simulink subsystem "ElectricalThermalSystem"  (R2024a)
settings: Solver=VariableStepAuto  StartTime=0.0  StopTime=10.0  RelTol=1e-3
undefined symbols (not defined in the file): EnvAirTemp, PlantThrEstCmpPwr, PlntThrAirBpt, PlntThrAirCond, PlntThrAirCp, PlntThrAirCpBpt, PlntThrAirPrand, PlntThrAirRho, PlntThrAirVisc, PlntThrBattDCFlwRatio, PlntThrBattJacLen, PlntThrChArea, PlntThrChDia, PlntThrCoolCond, PlntThrCoolCp, PlntThrCoolCpBpt, PlntThrCoolPrand, PlntThrCoolRho, PlntThrCoolVisc, PlntThrDCJacLen, PlntThrEMJacLen, PlntThrEstCOPLut, PlntThrEstDTLut, PlntThrHeaterMaxPwr, PlntThrPmpDisp, PlntThrPmpHeadP, PlntThrPmpMaxSpd, PlntThrPmpMechEff, PlntThrPmpVolEff, PlntThrRadAirArea, PlntThrRadAirDh, PlntThrRadFanAreaFlw, PlntThrRadFlwCoef, PlntThrRadGapHeight, PlntThrRadLength, PlntThrRadNTubes, PlntThrRadTubeDh, PlntThrRadTubeHeight, PlntThrRadWidth
libraries: autolibutils x45
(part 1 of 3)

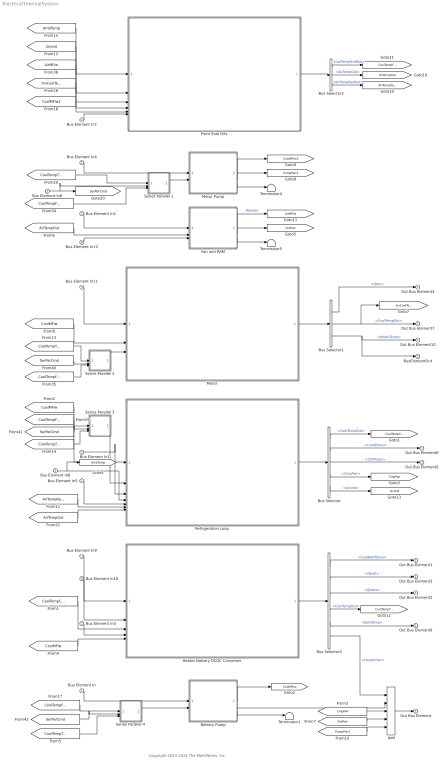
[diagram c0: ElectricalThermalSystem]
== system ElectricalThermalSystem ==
  note: Copyright 2023-2024 The MathWorks, Inc.
  Bus Element In{,1..7} (8 alike) : Inport
  Bus Element In8 : Inport  Port=2
  Bus Element In9 : Inport  Port=3
  Bus Element In10 : Inport  Port=4
  Bus Element In11 : Inport  Port=5
  Bus Element In12 : Inport  Port=6
  Add : Sum  Inputs=+++++
  Battery Pump : Subsystem  mask{DispAng=PlntThrPmpDisp, MaxSpd=PlntThrPmpMaxSpd, VolEff=PlntThrPmpVolEff, MechEff=PlntThrPmpMechEff, HeadP=PlntThrPmpHeadP}
      mask prompts: DispAng "Displacement per revolution, DispAng [L/rev]"; MaxSpd "Max angular speed, MaxSpd [rpm]"; VolEff "Volumetric efficiency, VolEff [-]"; MechEff "Mechanical efficiency, MechEff [-]"; HeadP "Pressure gain, HeadP [Pa]"
  Bus Selector : BusSelector  OutputSignals=CoolTempOut,CondPress,ChlrPress,CmpPwr,Qcond
  Bus Selector1 : BusSelector  OutputSignals=Qem,CoolTempOut,MotorTemp
  Bus Selector2 : BusSelector  OutputSignals=CoolTempFrmRad,AirTempOut,AirTempRadOut
  Bus Selector3 : BusSelector  OutputSignals=CoolBattTemp,Qbatt,Qpwre,CoolTempOut,BattTemp,HeaterPwr
  Fan and RAM : Subsystem  mask{DispAng=PlntThrPmpDisp, MaxSpd=PlntThrPmpMaxSpd, VolEff=PlntThrPmpVolEff, MechEff=PlntThrPmpMechEff, HeadP=PlntThrPmpHeadP}
      mask prompts: DispAng "Displacement per revolution, DispAng [L/rev]"; MaxSpd "Max angular speed, MaxSpd [rpm]"; VolEff "Volumetric efficiency, VolEff [-]"; MechEff "Mechanical efficiency, MechEff [-]"; HeadP "Pressure gain, HeadP [Pa]"
  Front Side HXs : Subsystem
  Heater Battery DCDC Converter : Subsystem
  Motor : Subsystem  Variant=on
  Motor Pump : Subsystem  mask{DispAng=PlntThrPmpDisp, MaxSpd=PlntThrPmpMaxSpd, VolEff=PlntThrPmpVolEff, MechEff=PlntThrPmpMechEff, HeadP=PlntThrPmpHeadP}
      mask prompts: DispAng "Displacement per revolution, DispAng [L/rev]"; MaxSpd "Max angular speed, MaxSpd [rpm]"; VolEff "Volumetric efficiency, VolEff [-]"; MechEff "Mechanical efficiency, MechEff [-]"; HeadP "Pressure gain, HeadP [Pa]"
  Refrigeration Loop : Subsystem
  Series Parallel 1 : Subsystem
  Series Parallel 2 : Subsystem
  Series Parallel 3 : Subsystem
  Series Parallel 4 : Subsystem
  Terminator1 : Terminator
  Terminator4 : Terminator
  Terminator5 : Terminator
  Out Bus Element{,1..7,9..10} (10 alike) : Outport
  BusElementOut : Outport
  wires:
  Bus Element In9/1 -> Heater Battery DCDC Converter/1(BattTemp)
  Bus Element In10/1 -> Heater Battery DCDC Converter/2(PwrETemp)
  Series Parallel 4/1(Out1) -> Battery Pump/2(FluidTemp)
  Series Parallel 3/1(Out1) -> Refrigeration Loop/2(CoolTempIn)
  Series Parallel 1/1(Out1) -> Motor Pump/2(FluidTemp)
  Motor/1(Info) -> Bus Selector1/1
  Series Parallel 2/1(Out1) -> Motor/3(CoolTempIn)
  [CoolMFlw] -> Motor/2(CoolMFlow)
  Bus Element In11/1 -> Motor/1(EMTemp)
  Bus Element In12/1 -> Fan and RAM/3(xdot)
  Bus Element In8/1 -> Refrigeration Loop/4(AmbTemp), [AmbTemp]
  [AirTempOut] -> Refrigeration Loop/7(AirTempCondOut)
  [AirTempRadOut] -> Refrigeration Loop/6(AirTempCondIn)
  Bus Selector2/3 -> [AirTempRadOut]  "<AirTempRadOut>"
  Bus Element In5/1 -> Refrigeration Loop/5(ByPCmd)
  Bus Element In7/1 -> Front Side HXs/6(ByPCmd)
  Bus Element In/1 -> Battery Pump/1(Cmd)
  Battery Pump/1(Mdot) -> [CoolMFlw]
  Battery Pump/3(Trq) -> Terminator1/1
  Bus Element In3/1 -> Heater Battery DCDC Converter/4(HeaterCmd)
  Heater Battery DCDC Converter/1(Bus Element Out) -> Bus Selector3/1
  Bus Selector3/1 -> Out Bus Element1/1  "<CoolBattTemp>"
  Bus Selector3/2 -> Out Bus Element3/1  "<Qbatt>"
  Bus Selector3/3 -> Out Bus Element2/1  "<Qpwre>"
  Bus Selector3/4 -> [CoolTempToRorC]  "<CoolTempOut>"
  [CoolMFlw] -> Refrigeration Loop/1(CoolMFlow)
  Bus Element In1/1 -> Refrigeration Loop/3(CmpCmd)
  [CoolTempChlrOut] -> Heater Battery DCDC Converter/3(CoolTempIn)
  Bus Selector/4 -> [CmpPwr]  "<CmpPwr>"
  Bus Selector/2 -> Out Bus Element6/1  "<CondPress>"
  Bus Selector/3 -> Out Bus Element5/1  "<ChlrPress>"
  Add/1 -> Out Bus Element/1
  [CoolMFlw] -> Heater Battery DCDC Converter/5(CoolMFlw)
  [AirTempOut] -> Fan and RAM/2(AirTemp)
  Bus Element In2/1 -> Fan and RAM/1(Cmd)
  Fan and RAM/1(Mdot) -> [AirMFlw]  "MdotAir"
  Fan and RAM/2(Pwr) -> [FanPwr]
  Fan and RAM/3(Trq) -> Terminator5/1
  Bus Selector1/1 -> Out Bus Element4/1  "<Qem>"
  Bus Selector1/2 -> Out Bus Element7/1, [InvCoolTempOut]  "<CoolTempOut>"
  Bus Element In4/1 -> Motor Pump/1(Cmd)
  Motor Pump/3(Trq) -> Terminator4/1
  Motor Pump/2(Pwr) -> [PumpPwr2]
  Motor Pump/1(Mdot) -> [CoolMFlw2]
  Bus Selector/5 -> [Qcond]  "<Qcond>"
  Refrigeration Loop/1(Out Bus Element) -> Bus Selector/1
  [AmbTemp] -> Front Side HXs/1(AmbTemp)
  [Qcond] -> Front Side HXs/2(Qcond)
  [AirMFlw] -> Front Side HXs/3(AirMFlw)
  [InvCoolTempOut] -> Front Side HXs/4(CoolTempToRad)
  Front Side HXs/1(Out Bus Element) -> Bus Selector2/1
  Bus Selector2/2 -> [AirTempOut]  "<AirTempOut>"
  [SerParCmd] -> Series Parallel 2/2(In2)
  [SerParCmd] -> Series Parallel 4/2(In2)
  [SerParCmd] -> Series Parallel 3/2(In2)
  Bus Element In6/1 -> [SerParCmd], Series Parallel 1/2(In2)
  [CoolMFlw2] -> Front Side HXs/5(CoolMFlw2)
  Bus Selector2/1 -> [CoolTempFrmRad]  "<CoolTempFrmRad>"
  Bus Selector/1 -> [CoolTempChlrOut]  "<CoolTempOut>"
  Bus Selector1/3 -> Out Bus Element10/1, BusElementOut/1  "<MotorTemp>"
  Bus Selector3/5 -> Out Bus Element9/1  "<BattTemp>"
  [PumpPwr2] -> Add/5
  [FanPwr] -> Add/4
  [CmpPwr] -> Add/3
  Battery Pump/2(Pwr) -> Add/2
  Bus Selector3/6 -> Add/1  "<HeaterPwr>"
  [CoolTempFrmRad] -> Series Parallel 3/1(In1)
  [CoolTempToRorC] -> Series Parallel 3/3(In3)
  [CoolTempToRorC] -> Series Parallel 2/1(In1)
  [CoolTempFrmRad] -> Series Parallel 2/3(In3)
  [CoolTempFrmRad] -> Series Parallel 4/1(In1)
  [CoolTempToRorC] -> Series Parallel 4/3(In3)
  [CoolTempToRorC] -> Series Parallel 1/1(In1)
  [CoolTempFrmRad] -> Series Parallel 1/3(In3)

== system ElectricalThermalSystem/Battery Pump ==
  Cmd : Inport
  FluidTemp : Inport  Port=2
  Density : Lookup_n-D  NumberOfTableDimensions=1  BreakpointsForDimension1=PlntThrCoolCpBpt  Table=PlntThrCoolRho  ExtrapMethod=Clip  UseLastTableValue=on  InternalRulePriority=Speed  RndMeth=Simplest
  Displ_LperRev : Constant  Value=DispAng  SampleTime=-1
  Gain : Gain  Gain=2*pi/60
  Gain1 : Gain  Gain=1/(1000*2*pi)
  LPF with IC1 : Subsystem  mask{wc=100, InitCond=0, dataType=off}
      mask prompts: wc "Cutoff frequency, wc [rad/s]"; InitCond "Initial condition, InitCond [same as u]"; dataType "Enforce same input data type"
  MaxSpd_rpm : Constant  Value=MaxSpd  SampleTime=-1
  MechanicalEfficiency : Constant  Value=MechEff  SampleTime=-1
  PressGain_Pa : Constant  Value=HeadP  SampleTime=-1
  Product : Product  Inputs=4
  Product1 : Product  Inputs=3
  Product2 : Product
  Product7 : Product
  Saturation : Saturate  UpperLimit=inf  LowerLimit=0
  VolumetricEfficiency : Constant  Value=VolEff  SampleTime=-1
  Mdot : Outport
  Pwr : Outport  Port=2
  Trq : Outport  Port=3
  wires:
  Saturation/1 -> Mdot/1
  LPF with IC1/1(y) -> Product7/2
  FluidTemp/1 -> Density/1
  VolumetricEfficiency/1 -> [VolEff]
  Density/1 -> Product/1
  MaxSpd_rpm/1 -> Gain/1
  Gain/1 -> Product7/1
  Displ_LperRev/1 -> Gain1/1
  Product7/1 -> [Spd]
  [Spd] -> Product/3
  [VolEff] -> Product/4
  MechanicalEfficiency/1 -> Product1/2
  [Spd] -> Product2/1
  PressGain_Pa/1 -> Product1/3
  Product1/1 -> Trq/1, Product2/2
  Gain1/1 -> Product1/1, Product/2
  Product/1 -> Saturation/1
  Cmd/1 -> LPF with IC1/1(u)
  Product2/1 -> Pwr/1

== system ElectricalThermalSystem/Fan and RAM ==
  Cmd : Inport
  AirTemp : Inport  Port=2
  xdot : Inport  Port=3
  Add : Sum
  Density : Lookup_n-D  NumberOfTableDimensions=1  BreakpointsForDimension1=PlntThrAirBpt  Table=PlntThrAirRho  ExtrapMethod=Clip  UseLastTableValue=on  InternalRulePriority=Speed  RndMeth=Simplest
  Displ_LperRev : Constant  Value=DispAng  SampleTime=-1
  Gain : Gain  Gain=PlntThrRadFanAreaFlw*PlntThrRadFlwCoef
  Gain1 : Gain  Gain=2*pi/60
  Gain2 : Gain  Gain=1/(1000*2*pi)
  LPF with IC1 : Subsystem  mask{wc=100, InitCond=0, dataType=off}
      mask prompts: wc "Cutoff frequency, wc [rad/s]"; InitCond "Initial condition, InitCond [same as u]"; dataType "Enforce same input data type"
  MaxSpd_rpm : Constant  Value=MaxSpd  SampleTime=-1
  MechanicalEfficiency : Constant  Value=MechEff  SampleTime=-1
  PressGain_Pa : Constant  Value=HeadP  SampleTime=-1
  Product : Product  Inputs=3
  Product1 : Product  Inputs=3
  Product2 : Product
  Product4 : Product
  Product7 : Product
  Saturation : Saturate  UpperLimit=inf  LowerLimit=0
  VolumetricEfficiency : Constant  Value=VolEff  SampleTime=-1
  Mdot : Outport
  Pwr : Outport  Port=2
  Trq : Outport  Port=3
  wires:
  Product4/1 -> Saturation/1
  Saturation/1 -> Mdot/1
  LPF with IC1/1(y) -> Product7/2
  AirTemp/1 -> Density/1
  Product/1 -> Add/2  "FanAir"
  xdot/1 -> Gain/1
  VolumetricEfficiency/1 -> [VolEff]
  Density/1 -> Product4/1
  MaxSpd_rpm/1 -> Gain1/1
  Gain1/1 -> Product7/1
  Displ_LperRev/1 -> Gain2/1
  Product7/1 -> [Spd]
  MechanicalEfficiency/1 -> Product1/2
  [Spd] -> Product2/1
  PressGain_Pa/1 -> Product1/3
  Product1/1 -> Trq/1, Product2/2
  Gain2/1 -> Product1/1, Product/1
  Cmd/1 -> LPF with IC1/1(u)
  Product2/1 -> Pwr/1
  [VolEff] -> Product/3
  [Spd] -> Product/2
  Add/1 -> Product4/2
  Gain/1 -> Add/1

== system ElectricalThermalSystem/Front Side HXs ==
  AmbTemp : Inport
  Qcond : Inport  Port=2
  AirMFlw : Inport  Port=3
  CoolTempToRad : Inport  Port=4
  CoolMFlw2 : Inport  Port=5
  ByPCmd : Inport  Port=6
  Condenser : Subsystem
  Radiator : Subsystem
  Out Bus Element{,1..3} (4 alike) : Outport
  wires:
  [AirMassFlw] -> Condenser/2(AirMassFlow)
  Radiator/2(Qrad) -> Out Bus Element2/1
  Radiator/1(CoolTempFrmRad) -> Out Bus Element/1
  ByPCmd/1 -> Radiator/5(ByPCmd)
  CoolMFlw2/1 -> Radiator/3(CoolMFlw)
  AmbTemp/1 -> Radiator/2(AmbTemp)
  CoolTempToRad/1 -> Radiator/1(CoolTempToRad)
  Radiator/3(AirTempOut) -> Out Bus Element3/1, Condenser/3(AirTempRadOut)
  Condenser/1(AirTempOut) -> Out Bus Element1/1
  Qcond/1 -> Condenser/1(Qcond)
  AirMFlw/1 -> [AirMassFlw], Radiator/4(MassFlow2)  "AirMassFlow"

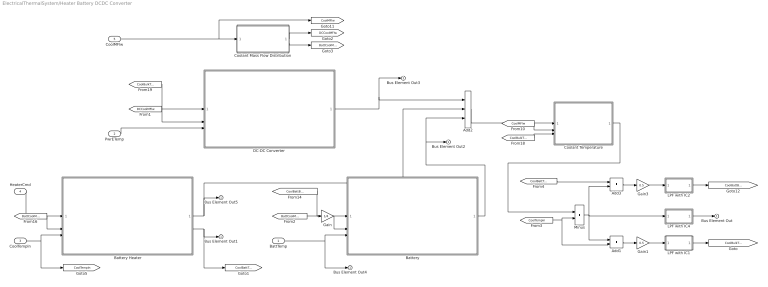
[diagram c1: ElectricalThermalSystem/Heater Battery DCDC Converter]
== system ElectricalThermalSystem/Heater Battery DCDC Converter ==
  BattTemp : Inport
  PwrETemp : Inport  Port=2
  CoolTempIn : Inport  Port=3
  HeaterCmd : Inport  Port=4
  CoolMFlw : Inport  Port=5
  Add1 : Sum
  Add2 : Sum  Inputs=+++
  Add3 : Sum
  Battery : Subsystem  mask{JacArea=PlntThrChArea, JacDia=PlntThrChDia, JacLen=PlntThrBattJacLen, JacHtArea=PlntThrBattJacLen*pi*PlntThrChDia}
      mask prompts: JacArea "Jacket cross section area, JacArea [m^2]"; JacDia "Jacket hydraulic diameter, JacDia [m]"; JacLen "Jacket length, JacLen [m]"; JacHtArea "Jacket heat transfer area, JacHtArea [m^2]"
  Battery Heater : Subsystem  mask{HtPwr=PlntThrHeaterMaxPwr}
      mask prompts: HtPwr "Maximum battery heater power, Gain [W]"
  Coolant Mass Flow Distribution : Subsystem  mask{MFlwRt=PlntThrBattDCFlwRatio}
      mask prompts: MFlwRt "Battery / DC-DC converter flow ratio, MFlwRt [-]"
  Coolant Temperature : Subsystem
  DC-DC Converter : Subsystem  mask{JacArea=PlntThrChArea, JacDia=PlntThrChDia, JacLen=PlntThrDCJacLen, JacHtArea=PlntThrDCJacLen*pi*PlntThrChDia}
      mask prompts: JacArea "Jacket cross section area, JacArea [m^2]"; JacDia "Jacket hydraulic diameter, JacDia [m]"; JacLen "Jacket length, JacLen [m]"; JacHtArea "Jacket heat transfer area, JacHtArea [m^2]"
  Gain : Gain  Gain=1/4
  Gain1 : Gain  Gain=0.5
  Gain3 : Gain  Gain=0.5
  LPF with IC1 : Subsystem  mask{wc=10, InitCond=EnvAirTemp, dataType=off}
      mask prompts: wc "Cutoff frequency, wc [rad/s]"; InitCond "Initial condition, InitCond [same as u]"; dataType "Enforce same input data type"
  LPF with IC2 : Subsystem  mask{wc=10, InitCond=EnvAirTemp, dataType=off}
      mask prompts: wc "Cutoff frequency, wc [rad/s]"; InitCond "Initial condition, InitCond [same as u]"; dataType "Enforce same input data type"
  LPF with IC4 : Subsystem  mask{wc=10, InitCond=EnvAirTemp, dataType=off}
      mask prompts: wc "Cutoff frequency, wc [rad/s]"; InitCond "Initial condition, InitCond [same as u]"; dataType "Enforce same input data type"
  Minus : Sum
  Bus Element Out{,1..5} (6 alike) : Outport
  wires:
  Battery Heater/1(Qheater) -> Add2/2, Bus Element Out5/1
  [CoolBattTempIn] -> Add3/1
  Battery Heater/2(CoolBattTemp) -> Bus Element Out1/1, [CoolBattTempIn]
  Coolant Temperature/1(DeltaTemp) -> Minus/1
  [CoolBulkTemp] -> Coolant Temperature/3(CoolBlkTemp)
  [CoolMFlw] -> Coolant Temperature/2(CoolMFlw)
  Add2/1 -> Coolant Temperature/1(Qsum)
  [BattCoolMFlw] -> Battery Heater/2(BattCoolMFlw)
  HeaterCmd/1 -> Battery Heater/1(HeaterCmd)
  PwrETemp/1 -> DC-DC Converter/3(PwrETemp)
  [DCCoolMFlw] -> DC-DC Converter/2(MassFlow)
  [CoolBulkTemp] -> DC-DC Converter/1(FluidTemp)
  DC-DC Converter/1(Qpwre) -> Add2/1, Bus Element Out3/1
  Gain/1 -> Battery/2(MassFlow)
  [CoolBattBulkTemp] -> Battery/1(FluidTemp)
  Battery/1(Qbatt) -> Bus Element Out2/1, Add2/3
  BattTemp/1 -> Bus Element Out4/1, Battery/3(BattTemp)
  Coolant Mass Flow Distribution/2(BattCoolMFlw) -> [BattCoolMFlw]
  Coolant Mass Flow Distribution/1(DCCoolMFlw) -> [DCCoolMFlw]
  [BattCoolMFlw] -> Gain/1
  LPF with IC4/1(y) -> Bus Element Out/1
  LPF with IC1/1(y) -> [CoolBulkTemp]
  Gain1/1 -> LPF with IC1/1(u)
  LPF with IC2/1(y) -> [CoolBattBulkTemp]
  Gain3/1 -> LPF with IC2/1(u)
  Add1/1 -> Gain1/1
  CoolTempIn/1 -> Battery Heater/3(CoolTempIn), [CoolTempIn]
  CoolMFlw/1 -> Coolant Mass Flow Distribution/1(CoolMFlw), [CoolMFlw]
  Add3/1 -> Gain3/1
  Minus/1 -> Add3/2, Add1/1, LPF with IC4/1(u)
  [CoolTempIn] -> Minus/2, Add1/2

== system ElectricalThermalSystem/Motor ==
  EMTemp : Inport
  CoolMFlow : Inport  Port=2
  CoolTempIn : Inport  Port=3
  FourEMs : Subsystem  VariantControl=PlntEMNum == 4
  OneEM : Subsystem  VariantControl=PlntEMNum == 1
  ThreeEMs : Subsystem  VariantControl=PlntEMNum == 3
  TwoEMs : Subsystem  VariantControl=PlntEMNum == 2
  Info : Outport

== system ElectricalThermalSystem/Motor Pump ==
  Cmd : Inport
  FluidTemp : Inport  Port=2
  Density : Lookup_n-D  NumberOfTableDimensions=1  BreakpointsForDimension1=PlntThrCoolCpBpt  Table=PlntThrCoolRho  ExtrapMethod=Clip  UseLastTableValue=on  InternalRulePriority=Speed  RndMeth=Simplest
  Displ_LperRev : Constant  Value=DispAng  SampleTime=-1
  Gain : Gain  Gain=2*pi/60
  Gain1 : Gain  Gain=1/(1000*2*pi)
  LPF with IC1 : Subsystem  mask{wc=100, InitCond=0, dataType=off}
      mask prompts: wc "Cutoff frequency, wc [rad/s]"; InitCond "Initial condition, InitCond [same as u]"; dataType "Enforce same input data type"
  MaxSpd_rpm : Constant  Value=MaxSpd  SampleTime=-1
  MechanicalEfficiency : Constant  Value=MechEff  SampleTime=-1
  PressGain_Pa : Constant  Value=HeadP  SampleTime=-1
  Product : Product  Inputs=4
  Product1 : Product  Inputs=3
  Product2 : Product
  Product7 : Product
  Saturation : Saturate  UpperLimit=inf  LowerLimit=0
  VolumetricEfficiency : Constant  Value=VolEff  SampleTime=-1
  Mdot : Outport
  Pwr : Outport  Port=2
  Trq : Outport  Port=3
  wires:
  Saturation/1 -> Mdot/1
  LPF with IC1/1(y) -> Product7/2
  FluidTemp/1 -> Density/1
  VolumetricEfficiency/1 -> [VolEff]
  Density/1 -> Product/1
  MaxSpd_rpm/1 -> Gain/1
  Gain/1 -> Product7/1
  Displ_LperRev/1 -> Gain1/1
  Product7/1 -> [Spd]
  [Spd] -> Product/3
  [VolEff] -> Product/4
  MechanicalEfficiency/1 -> Product1/2
  [Spd] -> Product2/1
  PressGain_Pa/1 -> Product1/3
  Product1/1 -> Trq/1, Product2/2
  Gain1/1 -> Product1/1, Product/2
  Product/1 -> Saturation/1
  Cmd/1 -> LPF with IC1/1(u)
  Product2/1 -> Pwr/1

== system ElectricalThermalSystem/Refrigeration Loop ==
  CoolMFlow : Inport
  CoolTempIn : Inport  Port=2
  CmpCmd : Inport  Port=3
  AmbTemp : Inport  Port=4
  ByPCmd : Inport  Port=5
  AirTempCondIn : Inport  Port=6
  AirTempCondOut : Inport  Port=7
  Chiller Coolant Temperature : Subsystem
  Chiller Pressure : Subsystem
  Condenser Pressure : Subsystem
  Heat-flow Rate and Power : Subsystem
  Out Bus Element{,1..4} (5 alike) : Outport
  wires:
  Heat-flow Rate and Power/3(Qchiller) -> Chiller Coolant Temperature/1(Qchiller)
  Heat-flow Rate and Power/2(CmpPwr) -> Out Bus Element3/1
  Heat-flow Rate and Power/1(Qcond) -> Out Bus Element4/1
  CmpCmd/1 -> Heat-flow Rate and Power/3(CmpCmd)
  [CoolTempIn] -> Heat-flow Rate and Power/2(CoolTempIn)
  AmbTemp/1 -> Heat-flow Rate and Power/1(AmbTemp)
  ByPCmd/1 -> Chiller Coolant Temperature/5(ByPCmd)
  CoolMFlow/1 -> Chiller Coolant Temperature/4(CoolMFlw)
  CoolTempIn/1 -> Chiller Coolant Temperature/3(CoolTempIn), [CoolTempIn]
  [CoolTempOut] -> Chiller Coolant Temperature/2(CoolTempOut)
  Chiller Coolant Temperature/1(CoolTOut) -> [CoolTempOut], Out Bus Element/1
  Chiller Pressure/1(ChlrPress) -> Out Bus Element2/1
  [CoolTempOut] -> Chiller Pressure/2(CoolTempOut)
  [CoolTempIn] -> Chiller Pressure/1(CoolTempIn)
  Condenser Pressure/1(CondPress) -> Out Bus Element1/1
  AirTempCondIn/1 -> Condenser Pressure/2(AirTempIn)
  AirTempCondOut/1 -> Condenser Pressure/1(AirTempOut)

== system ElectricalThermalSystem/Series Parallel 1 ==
  In1 : Inport
  In2 : Inport  Port=2
  In3 : Inport  Port=3
  Series Parallel : Switch  Criteria=u2 > Threshold  Threshold=0.5
  Out1 : Outport
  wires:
  In3/1 -> Series Parallel/3
  In2/1 -> Series Parallel/2
  In1/1 -> Series Parallel/1
  Series Parallel/1 -> Out1/1

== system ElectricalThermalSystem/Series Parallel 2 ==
  In1 : Inport
  In2 : Inport  Port=2
  In3 : Inport  Port=3
  Series Parallel : Switch  Criteria=u2 > Threshold  Threshold=0.5
  Out1 : Outport
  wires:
  In3/1 -> Series Parallel/3
  In2/1 -> Series Parallel/2
  In1/1 -> Series Parallel/1
  Series Parallel/1 -> Out1/1

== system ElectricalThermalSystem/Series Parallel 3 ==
  In1 : Inport
  In2 : Inport  Port=2
  In3 : Inport  Port=3
  Series Parallel : Switch  Criteria=u2 > Threshold  Threshold=0.5
  Out1 : Outport
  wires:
  In3/1 -> Series Parallel/3
  In2/1 -> Series Parallel/2
  In1/1 -> Series Parallel/1
  Series Parallel/1 -> Out1/1

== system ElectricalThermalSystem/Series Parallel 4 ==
  In1 : Inport
  In2 : Inport  Port=2
  In3 : Inport  Port=3
  Series Parallel : Switch  Criteria=u2 > Threshold  Threshold=0.5
  Out1 : Outport
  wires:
  In3/1 -> Series Parallel/3
  In2/1 -> Series Parallel/2
  In1/1 -> Series Parallel/1
  Series Parallel/1 -> Out1/1

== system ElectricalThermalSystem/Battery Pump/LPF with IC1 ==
  u : Inport
  Cont LPF IC : autolibutils/Cont LPF IC  wc=wc  aMode=1  dataType=off
  Initial Condition : Constant  Value=InitCond  SampleTime=-1
  y : Outport
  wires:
  Cont LPF IC/1 -> y/1
  u/1 -> Cont LPF IC/1
  Initial Condition/1 -> Cont LPF IC/2

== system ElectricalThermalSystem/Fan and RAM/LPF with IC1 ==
  u : Inport
  Cont LPF IC : autolibutils/Cont LPF IC  wc=wc  aMode=1  dataType=off
  Initial Condition : Constant  Value=InitCond  SampleTime=-1
  y : Outport
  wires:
  Cont LPF IC/1 -> y/1
  u/1 -> Cont LPF IC/1
  Initial Condition/1 -> Cont LPF IC/2

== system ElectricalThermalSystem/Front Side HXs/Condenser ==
  Qcond : Inport
  AirMassFlow : Inport  Port=2
  AirTempRadOut : Inport  Port=3
  Add2 : Sum
  Add3 : Sum
  Gain4 : Gain  Gain=0.5
  LPF with IC2 : Subsystem  mask{wc=10, InitCond=EnvAirTemp, dataType=off}
      mask prompts: wc "Cutoff frequency, wc [rad/s]"; InitCond "Initial condition, InitCond [same as u]"; dataType "Enforce same input data type"
  Product4 : Product  Inputs=*/
  Product7 : Product
  Specific Heat Air 1 : Lookup_n-D  NumberOfTableDimensions=1  BreakpointsForDimension1=PlntThrAirCpBpt  Table=PlntThrAirCp  ExtrapMethod=Clip  UseLastTableValue=on  InternalRulePriority=Speed  RndMeth=Simplest
  div0protect - abs poly3 : autolibutils/div0protect - abs poly  thresh=.001  aMode=1
  AirTempOut : Outport
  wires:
  AirMassFlow/1 -> Product7/1
  Qcond/1 -> Product4/1
  AirTempRadOut/1 -> Add3/1, [AirTempRadOut]
  Product7/1 -> div0protect - abs poly3/1
  [AirTempOut] -> Add3/2
  Add2/1 -> LPF with IC2/1(u)
  Add3/1 -> Gain4/1
  div0protect - abs poly3/1 -> Product4/2
  Product4/1 -> Add2/2
  Specific Heat Air 1/1 -> Product7/2
  LPF with IC2/1(y) -> [AirTempOut], AirTempOut/1
  Gain4/1 -> Specific Heat Air 1/1
  [AirTempRadOut] -> Add2/1

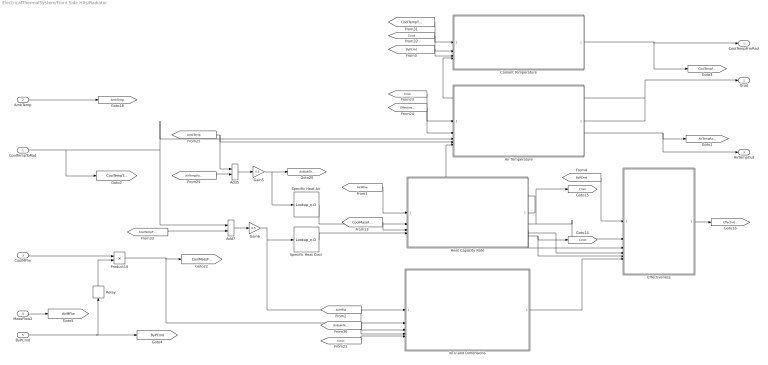
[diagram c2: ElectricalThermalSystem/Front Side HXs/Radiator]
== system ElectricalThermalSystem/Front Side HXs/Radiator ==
  CoolTempToRad : Inport
  AmbTemp : Inport  Port=2
  CoolMFlw : Inport  Port=3
  MassFlow2 : Inport  Port=4
  ByPCmd : Inport  Port=5
  Add5 : Sum
  Add7 : Sum
  Air Temperature : Subsystem
  Coolant Temperature : Subsystem
  Effectiveness : Subsystem
  Gain5 : Gain  Gain=0.5
  Gain6 : Gain  Gain=0.5
  Heat Capacity Rate : Subsystem
  NTU and Dimensions : Subsystem  mask{NTubes=PlntThrRadNTubes, DhCool=PlntThrRadTubeDh, RadLen=PlntThrRadLength, RadWid=PlntThrRadWidth, DhAir=PlntThrRadAirDh, AcCool=PlntThrRadWidth*PlntThrRadTubeHeight, AcAir=PlntThrRadLength*PlntThrRadGapHeight*0.9}
      mask prompts: NTubes "Number of tubes, [-]"; DhCool "Hydraulic diameter coolant side, DhCool [m]"; RadLen "Radiator length, RadLen"; RadWid "Radiator width, RadWid"; DhAir "Hydraulic diameter air side, DhAir [m]"; AcCool "Cross-sectional area coolant side, AcCool [m^2]"; AcAir "Cross-sectional area air side, AcAir"
  Product10 : Product
  Relay : Relay  OnSwitchValue=0.5  OffSwitchValue=0.5  OnOutputValue=eps  OffOutputValue=1
  Specific Heat Air : Lookup_n-D  NumberOfTableDimensions=1  BreakpointsForDimension1=PlntThrAirCpBpt  Table=PlntThrAirCp  ExtrapMethod=Clip  UseLastTableValue=on  InternalRulePriority=Speed  RndMeth=Simplest
  Specific Heat Cool : Lookup_n-D  NumberOfTableDimensions=1  BreakpointsForDimension1=PlntThrCoolCpBpt  Table=PlntThrCoolCp  ExtrapMethod=Clip  UseLastTableValue=on  InternalRulePriority=Speed  RndMeth=Simplest
  CoolTempFrmRad : Outport
  Qrad : Outport  Port=2
  AirTempOut : Outport  Port=3
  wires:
  [ByPCmd] -> Coolant Temperature/3(ByPCmd)
  Heat Capacity Rate/1(Cair) -> Air Temperature/5(Cair)
  [Effectiveness] -> Air Temperature/2(Effectiveness)
  [Cmin] -> Air Temperature/1(Cmin)
  Air Temperature/1(Qrad) -> Qrad/1, Coolant Temperature/4(Qrad)
  Air Temperature/2(AirTempOut) -> [AirTempRadOut], AirTempOut/1
  [Ccool] -> Coolant Temperature/2(Ccool)
  [CoolTempToRad] -> Coolant Temperature/1(CoolTempIn)
  Coolant Temperature/1(CoolTempOut) -> [CoolTempFrmRad], CoolTempFrmRad/1
  Effectiveness/1(Effectiveness) -> [Effectiveness]
  NTU and Dimensions/1(NTU) -> Effectiveness/6(NTU)
  Heat Capacity Rate/5(Ccool) -> [Ccool], Effectiveness/5(Ccool)
  Heat Capacity Rate/4(Cmax) -> Effectiveness/4(Cmax)
  Heat Capacity Rate/3(Cratio) -> Effectiveness/3(CminCmax)
  [ByPCmd] -> Effectiveness/1(ByPCmd)
  Specific Heat Cool/1 -> Heat Capacity Rate/4(CpCool)
  [CoolMassFlw] -> Heat Capacity Rate/3(CoolMFlw)
  Specific Heat Air/1 -> Heat Capacity Rate/2(CpAir)
  [AirMFlw] -> Heat Capacity Rate/1(AirMassFlw)
  Heat Capacity Rate/2(Cmin) -> [Cmin], Effectiveness/2(Cmin)
  [AirMFlw] -> NTU and Dimensions/3(MassFlow2)
  MassFlow2/1 -> [AirMFlw]
  Add7/1 -> Gain6/1
  Relay/1 -> Product10/2
  Gain5/1 -> [AirBulkTemp], Specific Heat Air/1
  Add5/1 -> Gain5/1
  [AirTempRadOut] -> Add5/2
  AmbTemp/1 -> [AmbTemp]
  [Cmin] -> NTU and Dimensions/5(Cmin)
  ByPCmd/1 -> Relay/1, [ByPCmd]
  [AmbTemp] -> Air Temperature/4(AirTempIn), Add5/1
  Product10/1 -> [CoolMassFlw], NTU and Dimensions/2(MassFlow1)
  CoolMFlw/1 -> Product10/1
  [CoolTempFrmRad] -> Add7/2
  [AirBulkTemp] -> NTU and Dimensions/4(FluidTemp2)
  Gain6/1 -> Specific Heat Cool/1, NTU and Dimensions/1(FluidTemp1)
  CoolTempToRad/1 -> [CoolTempToRad], Add7/1, Air Temperature/3(CoolTempIn)

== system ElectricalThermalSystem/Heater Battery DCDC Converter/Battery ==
  FluidTemp : Inport
  MassFlow : Inport  Port=2
  BattTemp : Inport  Port=3
  Constant3 : Constant  Value=JacHtArea  SampleTime=-1
  Constant6 : Constant  Value=JacDia  SampleTime=-1
  Constant7 : Constant  Value=JacArea  SampleTime=-1
  Constant8 : Constant  Value=JacLen  SampleTime=-1
  HTC Estimator Batt : Subsystem
  Heat-flow Rate : Subsystem
  Qbatt : Outport
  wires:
  Heat-flow Rate/1(Qbatt) -> Qbatt/1
  FluidTemp/1 -> HTC Estimator Batt/1(FluidTemp), Heat-flow Rate/4(CoolBlkTemp)
  BattTemp/1 -> Heat-flow Rate/3(BattTemp)
  Constant3/1 -> Heat-flow Rate/2(JacHtArea)
  HTC Estimator Batt/1(HTC) -> Heat-flow Rate/1(HTC)
  MassFlow/1 -> HTC Estimator Batt/2(MassFlow)
  Constant6/1 -> HTC Estimator Batt/4(HydDia)
  Constant8/1 -> HTC Estimator Batt/5(TubLen)
  Constant7/1 -> HTC Estimator Batt/3(CrossA)

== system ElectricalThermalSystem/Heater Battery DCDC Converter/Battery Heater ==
  HeaterCmd : Inport
  BattCoolMFlw : Inport  Port=2
  CoolTempIn : Inport  Port=3
  Add : Sum
  Add4 : Sum
  Divide1 : Product  Inputs=*/
  Gain4 : Gain  Gain=0.5
  LPF with IC3 : Subsystem  mask{wc=10, InitCond=EnvAirTemp, dataType=off}
      mask prompts: wc "Cutoff frequency, wc [rad/s]"; InitCond "Initial condition, InitCond [same as u]"; dataType "Enforce same input data type"
  Max Heat : Gain  Gain=HtPwr
  Product : Product
  Specific Heat1 : Lookup_n-D  NumberOfTableDimensions=1  BreakpointsForDimension1=PlntThrCoolCpBpt  Table=PlntThrCoolCp  ExtrapMethod=Clip  UseLastTableValue=on  InternalRulePriority=Speed  RndMeth=Simplest
  div0protect - abs poly1 : autolibutils/div0protect - abs poly  thresh=.001  aMode=1
  Qheater : Outport
  CoolBattTemp : Outport  Port=2
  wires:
  LPF with IC3/1(y) -> CoolBattTemp/1, [CoolBattTempIn]
  Add/1 -> LPF with IC3/1(u)
  HeaterCmd/1 -> Max Heat/1
  [CoolBattTempIn] -> Add4/1
  BattCoolMFlw/1 -> Product/1
  div0protect - abs poly1/1 -> Divide1/2
  Max Heat/1 -> Divide1/1, Qheater/1
  Add4/1 -> Gain4/1
  CoolTempIn/1 -> Add4/2, Add/2
  Product/1 -> div0protect - abs poly1/1
  Specific Heat1/1 -> Product/2
  Divide1/1 -> Add/1
  Gain4/1 -> Specific Heat1/1

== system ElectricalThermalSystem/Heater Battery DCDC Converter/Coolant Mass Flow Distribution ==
  CoolMFlw : Inport
  Gain2 : Gain  Gain=MFlwRt
  Minus1 : Sum  Inputs=+-
  DCCoolMFlw : Outport
  BattCoolMFlw : Outport  Port=2
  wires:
  Minus1/1 -> DCCoolMFlw/1
  CoolMFlw/1 -> Gain2/1, Minus1/1
  Gain2/1 -> Minus1/2, BattCoolMFlw/1

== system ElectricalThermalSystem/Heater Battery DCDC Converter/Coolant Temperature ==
  Qsum : Inport
  CoolMFlw : Inport  Port=2
  CoolBlkTemp : Inport  Port=3
  Divide : Product  Inputs=*/
  Product3 : Product
  Specific Heat : Lookup_n-D  NumberOfTableDimensions=1  BreakpointsForDimension1=PlntThrCoolCpBpt  Table=PlntThrCoolCp  ExtrapMethod=Clip  UseLastTableValue=on  InternalRulePriority=Speed  RndMeth=Simplest
  div0protect - abs poly4 : autolibutils/div0protect - abs poly  thresh=.001  aMode=1
  DeltaTemp : Outport
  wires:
  Divide/1 -> DeltaTemp/1
  CoolBlkTemp/1 -> Specific Heat/1
  Qsum/1 -> Divide/1
  CoolMFlw/1 -> Product3/1
  div0protect - abs poly4/1 -> Divide/2
  Product3/1 -> div0protect - abs poly4/1
  Specific Heat/1 -> Product3/2

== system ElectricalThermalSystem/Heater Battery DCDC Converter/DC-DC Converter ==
  FluidTemp : Inport
  MassFlow : Inport  Port=2
  PwrETemp : Inport  Port=3
  Constant : Constant  Value=JacDia  SampleTime=-1
  Constant2 : Constant  Value=JacHtArea  SampleTime=-1
  Constant4 : Constant  Value=JacArea  SampleTime=-1
  Constant5 : Constant  Value=JacLen  SampleTime=-1
  HTC Estimator DCDC : Subsystem
  Heat-flow Rate : Subsystem
  Qpwre : Outport
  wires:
  Heat-flow Rate/1(Qpwre) -> Qpwre/1
  FluidTemp/1 -> HTC Estimator DCDC/1(FluidTemp), Heat-flow Rate/4(CoolBlkTemp)
  Constant2/1 -> Heat-flow Rate/3(JacArea)
  PwrETemp/1 -> Heat-flow Rate/2(PwrETemp)
  HTC Estimator DCDC/1(HTC) -> Heat-flow Rate/1(HTC)
  MassFlow/1 -> HTC Estimator DCDC/2(MassFlow)
  Constant4/1 -> HTC Estimator DCDC/3(CrossA)
  Constant5/1 -> HTC Estimator DCDC/5(TubLen)
  Constant/1 -> HTC Estimator DCDC/4(HydDia)

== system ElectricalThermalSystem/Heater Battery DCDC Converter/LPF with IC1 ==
  u : Inport
  Cont LPF IC : autolibutils/Cont LPF IC  wc=wc  aMode=1  dataType=off
  Initial Condition : Constant  Value=InitCond  SampleTime=-1
  y : Outport
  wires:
  Cont LPF IC/1 -> y/1
  u/1 -> Cont LPF IC/1
  Initial Condition/1 -> Cont LPF IC/2

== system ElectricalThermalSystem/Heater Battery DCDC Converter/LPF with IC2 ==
  u : Inport
  Cont LPF IC : autolibutils/Cont LPF IC  wc=wc  aMode=1  dataType=off
  Initial Condition : Constant  Value=InitCond  SampleTime=-1
  y : Outport
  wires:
  Cont LPF IC/1 -> y/1
  u/1 -> Cont LPF IC/1
  Initial Condition/1 -> Cont LPF IC/2

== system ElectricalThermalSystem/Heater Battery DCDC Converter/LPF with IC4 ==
  u : Inport
  Cont LPF IC : autolibutils/Cont LPF IC  wc=wc  aMode=1  dataType=off
  Initial Condition : Constant  Value=InitCond  SampleTime=-1
  y : Outport
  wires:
  Cont LPF IC/1 -> y/1
  u/1 -> Cont LPF IC/1
  Initial Condition/1 -> Cont LPF IC/2

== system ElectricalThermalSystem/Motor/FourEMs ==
  EMTemp : Inport
  CoolMFlow : Inport  Port=2
  CoolTempIn : Inport  Port=3
  EM1 : Subsystem  mask{JacArea=PlntThrChArea, JacDia=PlntThrChDia, JacLen=PlntThrEMJacLen, JacHtArea=PlntThrEMJacLen*pi*PlntThrChDia}
      mask prompts: JacArea "Jacket cross section area, JacArea [m^2]"; JacDia "Jacket hydraulic diameter, JacDia [m]"; JacLen "Jacket length, JacLen [m]"; JacHtArea "Jacket heat transfer area, JacHtArea [m^2]"
  EM2 : Subsystem  mask{JacArea=PlntThrChArea, JacDia=PlntThrChDia, JacLen=PlntThrEMJacLen, JacHtArea=PlntThrEMJacLen*pi*PlntThrChDia}
      mask prompts: JacArea "Jacket cross section area, JacArea [m^2]"; JacDia "Jacket hydraulic diameter, JacDia [m]"; JacLen "Jacket length, JacLen [m]"; JacHtArea "Jacket heat transfer area, JacHtArea [m^2]"
  EM3 : Subsystem  mask{JacArea=PlntThrChArea, JacDia=PlntThrChDia, JacLen=PlntThrEMJacLen, JacHtArea=PlntThrEMJacLen*pi*PlntThrChDia}
      mask prompts: JacArea "Jacket cross section area, JacArea [m^2]"; JacDia "Jacket hydraulic diameter, JacDia [m]"; JacLen "Jacket length, JacLen [m]"; JacHtArea "Jacket heat transfer area, JacHtArea [m^2]"
  EM4 : Subsystem  mask{JacArea=PlntThrChArea, JacDia=PlntThrChDia, JacLen=PlntThrEMJacLen, JacHtArea=PlntThrEMJacLen*pi*PlntThrChDia}
      mask prompts: JacArea "Jacket cross section area, JacArea [m^2]"; JacDia "Jacket hydraulic diameter, JacDia [m]"; JacLen "Jacket length, JacLen [m]"; JacHtArea "Jacket heat transfer area, JacHtArea [m^2]"
  Max of Elements : MinMax  Function=max
  Vector Concatenate : Concatenate  NumInputs=4
  Bus Element Out3 : Outport
  Bus Element Out1 : Outport
  Bus Element Out4 : Outport
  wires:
  EM4/1(Qem) -> Vector Concatenate/4
  [EMTemp] -> EM4/3(EMTemp)
  [MassFlow] -> EM4/2(CoolMFlow)
  EM3/2(CoolTempOut) -> EM4/1(CoolTempIn)
  EM4/2(CoolTempOut) -> Bus Element Out1/1
  EM3/1(Qem) -> Vector Concatenate/3
  [EMTemp] -> EM3/3(EMTemp)
  [MassFlow] -> EM3/2(CoolMFlow)
  EM2/2(CoolTempOut) -> EM3/1(CoolTempIn)
  [EMTemp] -> EM2/3(EMTemp)
  [MassFlow] -> EM2/2(CoolMFlow)
  Max of Elements/1 -> Bus Element Out4/1
  Vector Concatenate/1 -> Bus Element Out3/1
  EM2/1(Qem) -> Vector Concatenate/2
  EM1/1(Qem) -> Vector Concatenate/1
  EM1/2(CoolTempOut) -> EM2/1(CoolTempIn)
  EMTemp/1 -> EM1/3(EMTemp), [EMTemp], Max of Elements/1
  CoolTempIn/1 -> EM1/1(CoolTempIn)
  CoolMFlow/1 -> EM1/2(CoolMFlow), [MassFlow]

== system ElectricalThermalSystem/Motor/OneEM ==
  EMTemp : Inport
  CoolMFlow : Inport  Port=2
  CoolTempIn : Inport  Port=3
  EM1 : Subsystem  mask{JacArea=PlntThrChArea, JacDia=PlntThrChDia, JacLen=PlntThrEMJacLen, JacHtArea=PlntThrEMJacLen*pi*PlntThrChDia}
      mask prompts: JacArea "Jacket cross section area, JacArea [m^2]"; JacDia "Jacket hydraulic diameter, JacDia [m]"; JacLen "Jacket length, JacLen [m]"; JacHtArea "Jacket heat transfer area, JacHtArea [m^2]"
  Bus Element Out3 : Outport
  Bus Element Out1 : Outport
  Bus Element Out4 : Outport
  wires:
  EM1/2(CoolTempOut) -> Bus Element Out1/1
  EMTemp/1 -> EM1/3(EMTemp), Bus Element Out4/1
  EM1/1(Qem) -> Bus Element Out3/1
  CoolTempIn/1 -> EM1/2(CoolTempIn)
  CoolMFlow/1 -> EM1/1(MassFlow)

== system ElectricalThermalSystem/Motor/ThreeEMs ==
  EMTemp : Inport
  CoolMFlow : Inport  Port=2
  CoolTempIn : Inport  Port=3
  EM1 : Subsystem  mask{JacArea=PlntThrChArea, JacDia=PlntThrChDia, JacLen=PlntThrEMJacLen, JacHtArea=PlntThrEMJacLen*pi*PlntThrChDia}
      mask prompts: JacArea "Jacket cross section area, JacArea [m^2]"; JacDia "Jacket hydraulic diameter, JacDia [m]"; JacLen "Jacket length, JacLen [m]"; JacHtArea "Jacket heat transfer area, JacHtArea [m^2]"
  EM2 : Subsystem  mask{JacArea=PlntThrChArea, JacDia=PlntThrChDia, JacLen=PlntThrEMJacLen, JacHtArea=PlntThrEMJacLen*pi*PlntThrChDia}
      mask prompts: JacArea "Jacket cross section area, JacArea [m^2]"; JacDia "Jacket hydraulic diameter, JacDia [m]"; JacLen "Jacket length, JacLen [m]"; JacHtArea "Jacket heat transfer area, JacHtArea [m^2]"
  EM3 : Subsystem  mask{JacArea=PlntThrChArea, JacDia=PlntThrChDia, JacLen=PlntThrEMJacLen, JacHtArea=PlntThrEMJacLen*pi*PlntThrChDia}
      mask prompts: JacArea "Jacket cross section area, JacArea [m^2]"; JacDia "Jacket hydraulic diameter, JacDia [m]"; JacLen "Jacket length, JacLen [m]"; JacHtArea "Jacket heat transfer area, JacHtArea [m^2]"
  Max of Elements : MinMax  Function=max
  Vector Concatenate : Concatenate  NumInputs=3
  Bus Element Out3 : Outport
  Bus Element Out1 : Outport
  Bus Element Out4 : Outport
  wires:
  EM3/1(Qem) -> Vector Concatenate/3
  [EMTemp] -> EM3/3(EMTemp)
  [MassFlow] -> EM3/2(CoolMFlow)
  EM2/2(CoolTempOut) -> EM3/1(CoolTempIn)
  EM3/2(CoolTempOut) -> Bus Element Out1/1
  [EMTemp] -> EM2/3(EMTemp)
  [MassFlow] -> EM2/2(CoolMFlow)
  Max of Elements/1 -> Bus Element Out4/1
  Vector Concatenate/1 -> Bus Element Out3/1
  EM2/1(Qem) -> Vector Concatenate/2
  EM1/1(Qem) -> Vector Concatenate/1
  EM1/2(CoolTempOut) -> EM2/1(CoolTempIn)
  EMTemp/1 -> EM1/3(EMTemp), [EMTemp], Max of Elements/1
  CoolTempIn/1 -> EM1/1(CoolTempIn)
  CoolMFlow/1 -> EM1/2(CoolMFlow), [MassFlow]

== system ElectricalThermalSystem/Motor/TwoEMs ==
  EMTemp : Inport
  CoolMFlow : Inport  Port=2
  CoolTempIn : Inport  Port=3
  EM1 : Subsystem  mask{JacArea=PlntThrChArea, JacDia=PlntThrChDia, JacLen=PlntThrEMJacLen, JacHtArea=PlntThrEMJacLen*pi*PlntThrChDia}
      mask prompts: JacArea "Jacket cross section area, JacArea [m^2]"; JacDia "Jacket hydraulic diameter, JacDia [m]"; JacLen "Jacket length, JacLen [m]"; JacHtArea "Jacket heat transfer area, JacHtArea [m^2]"
  EM2 : Subsystem  mask{JacArea=PlntThrChArea, JacDia=PlntThrChDia, JacLen=PlntThrEMJacLen, JacHtArea=PlntThrEMJacLen*pi*PlntThrChDia}
      mask prompts: JacArea "Jacket cross section area, JacArea [m^2]"; JacDia "Jacket hydraulic diameter, JacDia [m]"; JacLen "Jacket length, JacLen [m]"; JacHtArea "Jacket heat transfer area, JacHtArea [m^2]"
  Max of Elements : MinMax  Function=max
  Vector Concatenate : Concatenate
  Bus Element Out3 : Outport
  Bus Element Out1 : Outport
  Bus Element Out4 : Outport
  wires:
  [EMTemp] -> EM2/3(EMTemp)
  [MassFlow] -> EM2/2(CoolMFlow)
  Max of Elements/1 -> Bus Element Out4/1
  Vector Concatenate/1 -> Bus Element Out3/1
  EM2/1(Qem) -> Vector Concatenate/2
  EM1/1(Qem) -> Vector Concatenate/1
  EM2/2(CoolTempOut) -> Bus Element Out1/1
  EM1/2(CoolTempOut) -> EM2/1(CoolTempIn)
  EMTemp/1 -> EM1/3(EMTemp), [EMTemp], Max of Elements/1
  CoolTempIn/1 -> EM1/1(CoolTempIn)
  CoolMFlow/1 -> EM1/2(CoolMFlow), [MassFlow]

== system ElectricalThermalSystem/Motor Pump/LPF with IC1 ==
  u : Inport
  Cont LPF IC : autolibutils/Cont LPF IC  wc=wc  aMode=1  dataType=off
  Initial Condition : Constant  Value=InitCond  SampleTime=-1
  y : Outport
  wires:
  Cont LPF IC/1 -> y/1
  u/1 -> Cont LPF IC/1
  Initial Condition/1 -> Cont LPF IC/2

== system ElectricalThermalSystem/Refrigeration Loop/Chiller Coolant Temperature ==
  Qchiller : Inport
  CoolTempOut : Inport  Port=2
  CoolTempIn : Inport  Port=3
  CoolMFlw : Inport  Port=4
  ByPCmd : Inport  Port=5
  Add : Sum
  Divide : Product  Inputs=*/
  Gain1 : Gain  Gain=0.5
  LPF with IC3 : Subsystem  mask{wc=10, InitCond=EnvAirTemp, dataType=off}
      mask prompts: wc "Cutoff frequency, wc [rad/s]"; InitCond "Initial condition, InitCond [same as u]"; dataType "Enforce same input data type"
  Minus : Sum
  Product : Product
  Specific Heat : Lookup_n-D  NumberOfTableDimensions=1  BreakpointsForDimension1=PlntThrCoolCpBpt  Table=PlntThrCoolCp  ExtrapMethod=Clip  UseLastTableValue=on  InternalRulePriority=Speed  RndMeth=Simplest
  Switch6 : Switch  Criteria=u2 > Threshold  Threshold=0.5
  div0protect - abs poly2 : autolibutils/div0protect - abs poly  thresh=.001  aMode=1
  CoolTOut : Outport
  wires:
  CoolMFlw/1 -> Product/2
  Qchiller/1 -> Divide/1
  Switch6/1 -> CoolTOut/1
  CoolTempOut/1 -> Add/1
  Product/1 -> div0protect - abs poly2/1
  Specific Heat/1 -> Product/1
  ByPCmd/1 -> Switch6/2
  Gain1/1 -> Specific Heat/1
  div0protect - abs poly2/1 -> Divide/2
  [CoolTempIn] -> Switch6/1, Minus/1
  LPF with IC3/1(y) -> Switch6/3
  Minus/1 -> LPF with IC3/1(u)
  Add/1 -> Gain1/1
  CoolTempIn/1 -> [CoolTempIn], Add/2
  Divide/1 -> Minus/2

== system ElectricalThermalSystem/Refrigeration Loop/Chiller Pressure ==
  CoolTempIn : Inport
  CoolTempOut : Inport  Port=2
  1-D Lookup Table2 : Lookup_n-D  NumberOfTableDimensions=1  BreakpointsForDimension1=[0 1 3 7]  Table=[0.65 0.45 0.3 0.3]  ExtrapMethod=Clip  UseLastTableValue=on  InternalRulePriority=Speed  RndMeth=Simplest
  Subtract3 : Sum  Inputs=+-
  ChlrPress : Outport
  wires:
  1-D Lookup Table2/1 -> ChlrPress/1
  CoolTempOut/1 -> Subtract3/2
  CoolTempIn/1 -> Subtract3/1
  Subtract3/1 -> 1-D Lookup Table2/1

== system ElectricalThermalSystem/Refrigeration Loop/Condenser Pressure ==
  AirTempOut : Inport
  AirTempIn : Inport  Port=2
  1-D Lookup Table1 : Lookup_n-D  NumberOfTableDimensions=1  BreakpointsForDimension1=[0 4.5 10 13 20]  Table=[1.3 1.3 1.53 1.62 1.7]  ExtrapMethod=Clip  UseLastTableValue=on  InternalRulePriority=Speed  RndMeth=Simplest
  Subtract1 : Sum  Inputs=+-
  CondPress : Outport
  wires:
  1-D Lookup Table1/1 -> CondPress/1
  AirTempIn/1 -> Subtract1/2
  AirTempOut/1 -> Subtract1/1
  Subtract1/1 -> 1-D Lookup Table1/1

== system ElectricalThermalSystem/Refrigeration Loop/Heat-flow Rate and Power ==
  AmbTemp : Inport
  CoolTempIn : Inport  Port=2
  CmpCmd : Inport  Port=3
  1-D Lookup Table : Lookup_n-D  NumberOfTableDimensions=1  BreakpointsForDimension1=PlntThrEstDTLut  Table=PlntThrEstCOPLut  ExtrapMethod=Clip  InternalRulePriority=Speed  RndMeth=Simplest
  Add1 : Sum
  Gain : Gain  Gain=-1
  LPF with IC1 : Subsystem  mask{wc=0.2, InitCond=0, dataType=off}
      mask prompts: wc "Cutoff frequency, wc [rad/s]"; InitCond "Initial condition, InitCond [same as u]"; dataType "Enforce same input data type"
  Power Chiller : Product
  Power Comp : Gain  Gain=PlantThrEstCmpPwr
  Signal Specification : SignalSpecification  Unit=kW
  Signal Specification1 : SignalSpecification  Unit=watt
  Subtract : Sum  Inputs=+-
  Unit Conversion : UnitConversion
  Qcond : Outport
  CmpPwr : Outport  Port=2
  Qchiller : Outport  Port=3
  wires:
  CmpCmd/1 -> LPF with IC1/1(u)
  Gain/1 -> Qchiller/1
  Add1/1 -> Qcond/1
  AmbTemp/1 -> Subtract/1
  Signal Specification1/1 -> Power Chiller/2, [CmpPwr], CmpPwr/1
  Power Comp/1 -> Signal Specification/1
  Signal Specification/1 -> Unit Conversion/1
  Power Chiller/1 -> Gain/1, Add1/2
  Subtract/1 -> 1-D Lookup Table/1
  [CmpPwr] -> Add1/1
  LPF with IC1/1(y) -> Power Comp/1
  1-D Lookup Table/1 -> Power Chiller/1
  CoolTempIn/1 -> Subtract/2
  Unit Conversion/1 -> Signal Specification1/1

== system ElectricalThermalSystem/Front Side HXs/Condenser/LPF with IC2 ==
  u : Inport
  Cont LPF IC : autolibutils/Cont LPF IC  wc=wc  aMode=1  dataType=off
  Initial Condition : Constant  Value=InitCond  SampleTime=-1
  y : Outport
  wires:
  Cont LPF IC/1 -> y/1
  u/1 -> Cont LPF IC/1
  Initial Condition/1 -> Cont LPF IC/2

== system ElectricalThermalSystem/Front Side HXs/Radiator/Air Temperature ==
  Cmin : Inport
  Effectiveness : Inport  Port=2
  CoolTempIn : Inport  Port=3
  AirTempIn : Inport  Port=4
  Cair : Inport  Port=5
  Add4 : Sum
  LPF with IC1 : Subsystem  mask{wc=10, InitCond=EnvAirTemp, dataType=off}
      mask prompts: wc "Cutoff frequency, wc [rad/s]"; InitCond "Initial condition, InitCond [same as u]"; dataType "Enforce same input data type"
  Product3 : Product  Inputs=3
  Product5 : Product  Inputs=*/
  Saturation1 : Saturate  UpperLimit=inf  LowerLimit=173.15
  Subtract : Sum  Inputs=+-
  div0protect - abs poly1 : autolibutils/div0protect - abs poly  thresh=.001  aMode=1
  Qrad : Outport
  AirTempOut : Outport  Port=2
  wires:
  [AirTempIn] -> Add4/1
  AirTempIn/1 -> Subtract/2, [AirTempIn]
  Effectiveness/1 -> Product3/2
  CoolTempIn/1 -> Subtract/1
  Cmin/1 -> Product3/1
  Product5/1 -> Add4/2
  LPF with IC1/1(y) -> AirTempOut/1
  Product3/1 -> Product5/1, Qrad/1
  div0protect - abs poly1/1 -> Product5/2
  Saturation1/1 -> LPF with IC1/1(u)
  Add4/1 -> Saturation1/1
  Cair/1 -> div0protect - abs poly1/1
  Subtract/1 -> Product3/3

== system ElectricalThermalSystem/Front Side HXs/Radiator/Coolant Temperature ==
  CoolTempIn : Inport
  Ccool : Inport  Port=2
  ByPCmd : Inport  Port=3
  Qrad : Inport  Port=4
  Add6 : Sum  Inputs=+-
  LPF Temperature : Subsystem  mask{wc=1, InitCond=EnvAirTemp, dataType=off}
      mask prompts: wc "Cutoff frequency, wc [rad/s]"; InitCond "Initial condition, InitCond [same as u]"; dataType "Enforce same input data type"
  Product6 : Product  Inputs=*/
  Saturation : Saturate  UpperLimit=inf  LowerLimit=173.15
  Switch5 : Switch  Criteria=u2 > Threshold  Threshold=0.5
  div0protect - abs poly : autolibutils/div0protect - abs poly  thresh=.001  aMode=1
  CoolTempOut : Outport
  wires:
  Ccool/1 -> div0protect - abs poly/1
  Qrad/1 -> Product6/1
  Saturation/1 -> Switch5/3
  div0protect - abs poly/1 -> Product6/2
  CoolTempIn/1 -> Switch5/1, Add6/1
  Product6/1 -> Add6/2
  LPF Temperature/1(y) -> CoolTempOut/1
  Switch5/1 -> LPF Temperature/1(u)
  Add6/1 -> Saturation/1
  ByPCmd/1 -> Switch5/2

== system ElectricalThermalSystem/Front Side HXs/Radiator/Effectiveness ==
  ByPCmd : Inport
  Cmin : Inport  Port=2
  CminCmax : Inport  Port=3
  Cmax : Inport  Port=4
  Ccool : Inport  Port=5
  NTU : Inport  Port=6
  Constant5 : Constant  SampleTime=-1
  Constant9 : Constant  Value=0  SampleTime=-1
  Effectiveness Calc : Fcn  Expr=(u(3)==u(5))*(1/u(2))*(1-exp(-u(2)*(1-exp(-u(4)))))+(u(1)==u(5))*(1-exp((-1/u(2))*(1-exp(-u(2)*u(4)))))
  Product2 : Product
  Switch1 : Switch  Criteria=u2 > Threshold  Threshold=0.5
  Vector Concatenate : Concatenate  NumInputs=5
  div0protect - abs poly5 : autolibutils/div0protect - abs poly  thresh=.001  aMode=1
  Effectiveness : Outport
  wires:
  CminCmax/1 -> div0protect - abs poly5/1
  div0protect - abs poly5/1 -> Vector Concatenate/2
  NTU/1 -> Vector Concatenate/4
  ByPCmd/1 -> Switch1/2
  Ccool/1 -> Vector Concatenate/5
  Cmin/1 -> Vector Concatenate/1
  Vector Concatenate/1 -> Effectiveness Calc/1
  Cmax/1 -> Vector Concatenate/3
  Effectiveness Calc/1 -> Product2/2
  Product2/1 -> Effectiveness/1
  Constant9/1 -> Switch1/1
  Constant5/1 -> Switch1/3
  Switch1/1 -> Product2/1

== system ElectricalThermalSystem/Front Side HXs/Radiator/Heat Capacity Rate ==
  AirMassFlw : Inport
  CpAir : Inport  Port=2
  CoolMFlw : Inport  Port=3
  CpCool : Inport  Port=4
  Divide2 : Product  Inputs=*/  RndMeth=Zero  SaturateOnIntegerOverflow=on
  Min : MinMax  Function=max  Inputs=2
  Min1 : MinMax  Inputs=2
  Product : Product
  Product1 : Product
  div0protect - abs poly2 : autolibutils/div0protect - abs poly  thresh=.001  aMode=1
  Cair : Outport
  Cmin : Outport  Port=2
  Cratio : Outport  Port=3
  Cmax : Outport  Port=4
  Ccool : Outport  Port=5
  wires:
  CoolMFlw/1 -> Product1/1
  AirMassFlw/1 -> Product/1
  CpCool/1 -> Product1/2
  Divide2/1 -> Cratio/1
  Product/1 -> Min/1, Min1/1, Cair/1
  div0protect - abs poly2/1 -> Divide2/2
  Min1/1 -> Divide2/1, Cmin/1
  CpAir/1 -> Product/2
  Min/1 -> div0protect - abs poly2/1, Cmax/1  "Cmax"
  [Ccool] -> Min1/2  "Ccool"
  Product1/1 -> Min/2, [Ccool], Ccool/1

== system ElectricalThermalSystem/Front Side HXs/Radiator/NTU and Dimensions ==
  FluidTemp1 : Inport
  MassFlow1 : Inport  Port=2
  MassFlow2 : Inport  Port=3
  FluidTemp2 : Inport  Port=4
  Cmin : Inport  Port=5
  Add : Sum
  Bias : Bias  Bias=1
  Constant : Constant  Value=NTubes  SampleTime=-1
  Constant1 : Constant  Value=DhCool  SampleTime=-1
  Constant2 : Constant  Value=RadWid  SampleTime=-1
  Constant4 : Constant  Value=DhAir  SampleTime=-1
  Constant6 : Constant  Value=RadLen  SampleTime=-1
  Constant7 : Constant  Value=AcCool  SampleTime=-1
  Constant8 : Constant  Value=AcAir  SampleTime=-1
  Divide : Product  Inputs=*/
  Divide1 : Product  Inputs=*/
  Divide3 : Product  Inputs=*/
  Gain : Gain  Gain=PlntThrRadAirArea
  Gain1 : Gain  Gain=PlntThrRadAirArea
  HTC Estimator Air : Subsystem
  HTC Estimator Coolant : Subsystem
  Math Function : Math  Operator=reciprocal
  Math Function1 : Math  Operator=reciprocal
  Math Function2 : Math  Operator=reciprocal
  div0protect - abs poly{1..5} (5 alike) : autolibutils/div0protect - abs poly  thresh=.001  aMode=1
  NTU : Outport
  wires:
  Math Function1/1 -> Add/2
  Math Function/1 -> Add/1
  div0protect - abs poly2/1 -> Math Function/1
  Gain/1 -> div0protect - abs poly2/1
  Gain1/1 -> div0protect - abs poly4/1
  div0protect - abs poly4/1 -> Math Function1/1
  Add/1 -> div0protect - abs poly5/1
  div0protect - abs poly5/1 -> Math Function2/1
  Math Function2/1 -> Divide3/1
  div0protect - abs poly1/1 -> Divide/2
  Cmin/1 -> div0protect - abs poly3/1
  div0protect - abs poly3/1 -> Divide3/2
  Divide3/1 -> NTU/1
  MassFlow2/1 -> Divide1/1
  Constant4/1 -> HTC Estimator Air/4(HydDia)
  Constant1/1 -> HTC Estimator Coolant/4(HydDia)
  HTC Estimator Air/1(HTC) -> Gain1/1
  Constant8/1 -> HTC Estimator Air/3(CrossA)
  Divide1/1 -> HTC Estimator Air/2(MassFlow)
  Constant7/1 -> HTC Estimator Coolant/3(CrossA)
  FluidTemp1/1 -> HTC Estimator Coolant/1(FluidTemp)
  Divide/1 -> HTC Estimator Coolant/2(MassFlow)
  FluidTemp2/1 -> HTC Estimator Air/1(FluidTemp)
  Bias/1 -> Divide1/2
  MassFlow1/1 -> Divide/1
  Constant/1 -> Bias/1, div0protect - abs poly1/1
  Constant6/1 -> HTC Estimator Coolant/5(TubLen)
  HTC Estimator Coolant/1(HTC) -> Gain/1
  Constant2/1 -> HTC Estimator Air/5(TubLen)

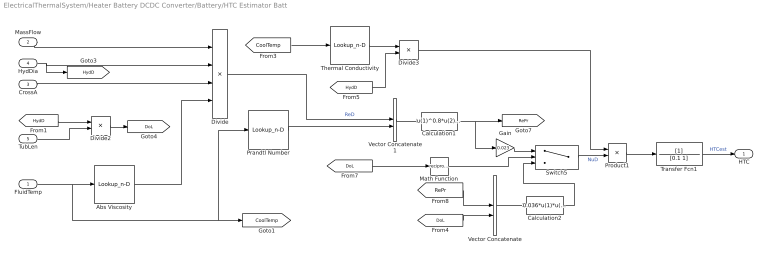
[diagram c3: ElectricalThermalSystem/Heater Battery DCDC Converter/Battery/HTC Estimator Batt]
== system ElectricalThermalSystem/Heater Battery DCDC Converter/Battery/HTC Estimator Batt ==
  FluidTemp : Inport
  MassFlow : Inport  Port=2
  CrossA : Inport  Port=3  OutMin=eps
  HydDia : Inport  Port=4
  TubLen : Inport  Port=5
  Abs Viscosity : Lookup_n-D  NumberOfTableDimensions=1  BreakpointsForDimension1=PlntThrCoolCpBpt  Table=PlntThrCoolVisc  ExtrapMethod=Clip  UseLastTableValue=on  InternalRulePriority=Speed  RndMeth=Simplest
  Calculation1 : Fcn  Expr=u(1)^0.8*u(2)^0.33
  Calculation2 : Fcn  Expr=0.036*u(1)*u(2)^0.055
  Divide : Product  Inputs=**//
  Divide2 : Product  Inputs=*/
  Divide3 : Product  Inputs=*/
  Gain : Gain  Gain=0.023
  Math Function : Math  Operator=reciprocal
  Prandtl Number : Lookup_n-D  NumberOfTableDimensions=1  BreakpointsForDimension1=PlntThrCoolCpBpt  Table=PlntThrCoolPrand  ExtrapMethod=Clip  UseLastTableValue=on  InternalRulePriority=Speed  RndMeth=Simplest
  Product1 : Product
  Switch5 : Switch  Threshold=400
  Thermal Conductivity : Lookup_n-D  NumberOfTableDimensions=1  BreakpointsForDimension1=PlntThrCoolCpBpt  Table=PlntThrCoolCond  ExtrapMethod=Clip  UseLastTableValue=on  InternalRulePriority=Speed  RndMeth=Simplest
  Transfer Fcn1 : TransferFcn  Denominator=[0.1 1]
  Vector Concatenate : Concatenate
  Vector Concatenate1 : Concatenate
  HTC : Outport
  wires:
  Product1/1 -> Transfer Fcn1/1
  Switch5/1 -> Product1/2  "NuD"
  Calculation2/1 -> Switch5/3
  Vector Concatenate/1 -> Calculation2/1
  [DoL] -> Vector Concatenate/2
  [RePr] -> Vector Concatenate/1
  Calculation1/1 -> Gain/1, [RePr]
  Gain/1 -> Switch5/1
  Divide3/1 -> Product1/1
  [HydD] -> Divide3/2
  Thermal Conductivity/1 -> Divide3/1
  Math Function/1 -> Switch5/2
  [DoL] -> Math Function/1
  Vector Concatenate1/1 -> Calculation1/1
  Prandtl Number/1 -> Vector Concatenate1/2
  Divide/1 -> Vector Concatenate1/1  "ReD"
  Abs Viscosity/1 -> Divide/4
  Divide2/1 -> [DoL]
  TubLen/1 -> Divide2/2
  [HydD] -> Divide2/1
  CrossA/1 -> Divide/3
  HydDia/1 -> Divide/2, [HydD]
  MassFlow/1 -> Divide/1
  [CoolTemp] -> Thermal Conductivity/1
  FluidTemp/1 -> Abs Viscosity/1, [CoolTemp], Prandtl Number/1
  Transfer Fcn1/1 -> HTC/1  "HTCest"
